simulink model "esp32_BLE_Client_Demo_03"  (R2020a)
settings: Solver=FixedStepDiscrete  StartTime=0.0  StopTime=10.0  RelTol=1e-3  EnableMultiTasking=on
undefined symbols (not defined in the file): BLE_demo, Client, CR, demo, Demo_03, ESP, esp32, esp32_BLE_Client_Demo_03_esp32_build_system, float, IDF, In1, In2, IP, Out1, Out2, Param1, r, SPP_BLE, targets, TCP, Trunk, uint32_t, waijung2
libraries: waijung2_utilities_lib x3, esp32_ble_lib x2, esp32_device_config_lib x1

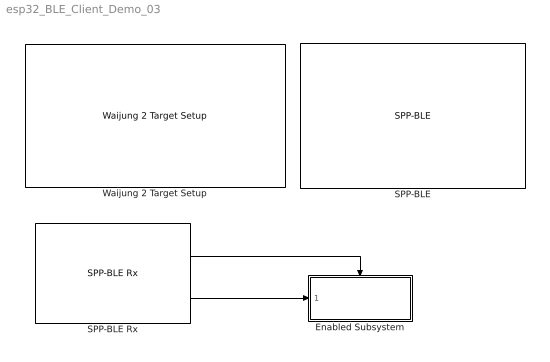
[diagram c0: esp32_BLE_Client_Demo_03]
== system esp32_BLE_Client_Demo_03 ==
  Enabled Subsystem : Subsystem  TreatAsAtomicUnit=on
  SPP-BLE : esp32_ble_lib/SPP-BLE  conf=Setup  spp=Client  ssid=BLE Server Demo 2  uartmodule=0  baudrate=115200  databits=8  parity=None  stopbit=1  txpin=32  rxpin=33  advanceoptions=on  rxbuffersize=256  txbuffersize=256  porttype_double=0  porttype_single=0  porttype_int8=0  porttype_uint8=0  porttype_int16=0  porttype_uint16=0  porttype_int32=0  porttype_uint32=2  asciiformat='Value=%1.2f'  tx_asciiterminator="CR (0x0D - \"\\r\")"  rx_asciiterminator="CR (0x0D - \"\\r\")"  buffersize=128  storagename=1  portpinstr=0  sampletime=-1  enablecustomportlabel=off  cinputportlabel=In1,In2  coutputportlabel=Out1,Out2  blockid=SPPBLE  inputporttype=[]  inputportwidth=[]  inputportlabel={}  outputporttype=[]  outputportwidth=[[]]  outputportlabel={}  compat=0  optionstring="[\"0\",\"115200\",\"Client\",\"BLE Server Demo 2\",\"256\",\"256\",\"Value=%1.2f\",\"\",\"\",\"UART_DATA_8_BITS\",\"UART_PARITY_DISABLE\",\"UART_STOP_BITS_1\",\"128\"]"  optionstring2="[\"float\"]"  MsgBufferSize=16
  SPP-BLE Rx : esp32_ble_lib/SPP-BLE Rx  conf=Rx  spp=Client  ssid=BLE SPP Server  uartmodule=0  databits=8  parity=None  stopbit=1  txpin=32  rxpin=33  advanceoptions=on  rxbuffersize=256  txbuffersize=256  porttype_double=0  porttype_single=0  porttype_int8=0  porttype_uint8=0  porttype_int16=0  porttype_uint16=0  porttype_int32=0  porttype_uint32=2  asciiformat='Joystick_Values=%s'  tx_asciiterminator="CR (0x0D - \"\\r\")"  rx_asciiterminator="CR (0x0D - \"\\r\")"  buffersize=128  storagename=1  portpinstr=0  sampletime=-1  enablecustomportlabel=off  cinputportlabel=In1,In2  coutputportlabel=Out1,Out2  blockid=SPPBLERx  inputporttype=[]  inputportwidth=[]  inputportlabel={}  outputporttype=[3 3]  outputportwidth=[1 64]  outputportlabel={'READY' 'string'}  compat=0  optionstring="[\"0\",\"\",\"Client\",\"BLE SPP Server\",\"256\",\"256\",\"Joystick_Values=%s\",\"0x0D\",\"1\",\"UART_DATA_8_BITS\",\"UART_PARITY_DISABLE\",\"UART_STOP_BITS_1\",\"128\"]"  optionstring2="[\"char *\"]"  rxdatatype='string'  MsgBufferSize=64
  Waijung 2 Target Setup : esp32_device_config_lib/Waijung 2 Target Setup  waijungversion=22.12a  toolchain=ESP-IDF  os=FreeRTOS  sampletime=-1  simulink_managebuildsystem=on  projectpath=E:\Trunk\waijung2\targets\esp32\demo\BLE_demo\SPP_BLE\Demo_03\Client\esp32_BLE_Client_Demo_03_esp32_build_system  espidfpath=C:\msys32\home\skris\esp\esp-idf  buildoptions=Deploy to hardware  blockid=Waijung2TargetSetup  target=ESP32  defaultstacksize=4086  basepriority=0  highestpriority=10  generate_baserate_task=on  tickrate=1000  esp32target=ESP32  esp32targetdef=esp32  esp32flashsize=4MB  esp32comport=COM3  esp32baudrate=115200  esp32advancedconfig=off  esp32partitiontable=Use default waijung2 partition table  esp32partitionpath=Browse the partition table  partitionname=partitions.csv  editpartition=on  custompartitiondata={'nvs','data','nvs','','0x6000','';'phy_init','data','phy','','0x1000','';'factory','app','factory','','1M',''}  reqblocks=default  esp32custompartition={'nvs','data','nvs','','0x6000','';'phy_init','data','phy','','0x1000','';'factory','app','factory','','1M',''}  cominterface=TCP/IP  uart_module=0  baudrate=115200  tx_pin=0  rx_pin=0  com_port=9  wifimode=WIFI AP  wifissid=esp32ssid  wifipassword=password  deviceip=192.168.1.10  targetgateway=192.168.1.1  targetnetmask=255.255.255.0  manualdns=on  targetdnsip=8.8.8.8  targetipport=256  targetipdef=0  targetmaskdef=0  targetgatewaydef=0  targetdnsipdef=0  hosttimeout=10  hostverbose=off
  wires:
  SPP-BLE Rx/1 -> Enabled Subsystem/Enable
  SPP-BLE Rx/2 -> Enabled Subsystem/1(In1)

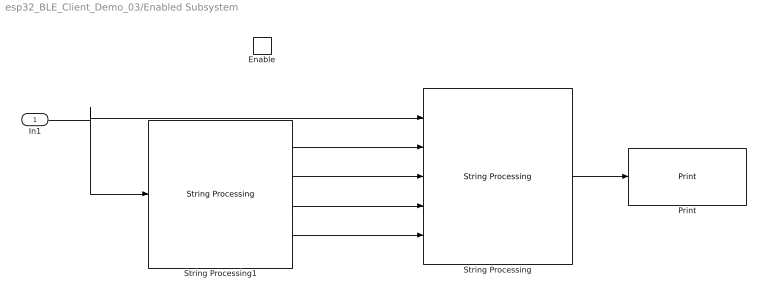
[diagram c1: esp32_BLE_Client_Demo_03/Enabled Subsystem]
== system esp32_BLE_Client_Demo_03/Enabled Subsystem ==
  In1 : Inport
  Enable : EnablePort
  Print : waijung2_utilities_lib/Print  printfcn=printf  strinput=Character Vector  sampletime=-1  blockid=EnabledSubsystemPrint  sampletimestr=2
  String Processing : waijung2_utilities_lib/String Processing  conf=processing  stringfunction=sprintf  stringformat='Raw values from the server:%s\nExtracted values:\nJS val 01: %u\nJS val 02: %u\nJS val 03: %u\nJS val 04: %u\n\n'  begindelimiter=''  enddelimiter=''  buffersize=128  enablestatus=off  use_pointer=off  pointer_list="\"\""  string_pointer=off  portpinstr=0  sampletime=-1  blockid=EnabledSubsystemStringProcessing  inputporttype=[3 -1 -1 -1 -1]  inputportwidth=[-1 1 1 1 1]  inputportlabel={'%s','%u','%u','%u','%u'}  outputporttype=[3]  outputportwidth=[128]  outputportlabel={'Output'}  compat=0  optionstring="[\"Param1\",\"Param1\"]"  datatypestring="[\"char *\",\"uint32_t\",\"uint32_t\",\"uint32_t\",\"uint32_t\"]"
  String Processing1 : waijung2_utilities_lib/String Processing  conf=processing  stringfunction=sscanf  stringformat='%u,%u,%u,%u'  begindelimiter=''  enddelimiter=''  buffersize=64  enablestatus=off  use_pointer=off  pointer_list="\"\""  string_pointer=off  portpinstr=0  sampletime=-1  blockid=EnabledSubsystemStringProcessing1  inputporttype=[3]  inputportwidth=[-1]  inputportlabel={'Input'}  outputporttype=[7 7 7 7]  outputportwidth=[1 1 1 1]  outputportlabel={'D1(uint32)','D2(uint32)','D3(uint32)','D4(uint32)'}  compat=0  optionstring="[\"Param1\",\"Param1\"]"  datatypestring="[\"uint32_t\",\"uint32_t\",\"uint32_t\",\"uint32_t\"]"
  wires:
  In1/1 -> String Processing1/1, String Processing/1
  String Processing/1 -> Print/1
  String Processing1/1 -> String Processing/2
  String Processing1/2 -> String Processing/3
  String Processing1/3 -> String Processing/4
  String Processing1/4 -> String Processing/5
